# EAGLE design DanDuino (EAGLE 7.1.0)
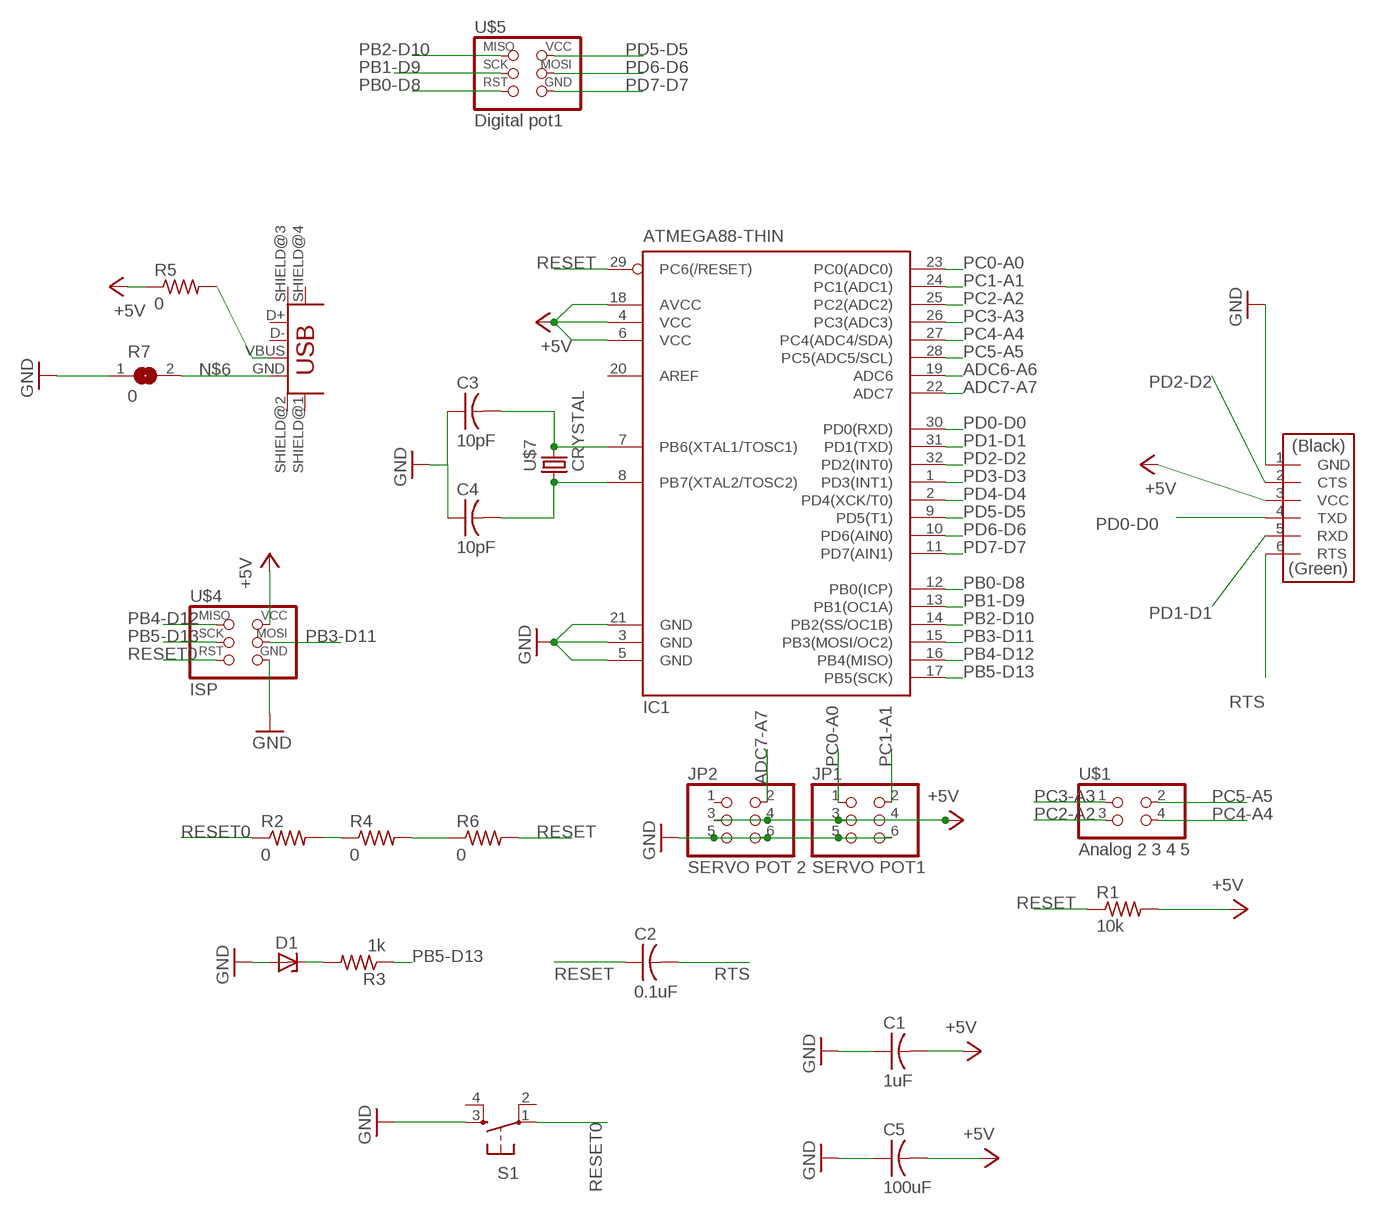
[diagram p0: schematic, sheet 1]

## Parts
C1  1uF  CAP-US1206FAB  [C1206FAB]
C2  0.1uF  CAP-US1206FAB  [C1206FAB]
C3  10pF  CAP-US1206FAB  [C1206FAB]
C4  10pF  CAP-US1206FAB  [C1206FAB]
C5  100uF  CAP-US1206FAB  [C1206FAB]
D1  ZENER_DIODESOD123  [SOD123]
IC1  ATMEGA88-THIN  [TQFP32-08THIN]
JP1  SERVO POT1  PINHD-2X3-SMD  [2X03SMD]
JP2  SERVO POT 2  PINHD-2X3-SMD  [2X03SMD]
R1  10k  RES-US1206FAB  [R1206FAB]
R2  0  RES-US1206FAB  [R1206FAB]
R3  1k  RES-US1206FAB  [R1206FAB]
R4  0  RES-US1206FAB  [R1206FAB]
R5  0  RES-US1206FAB  [R1206FAB]
R6  0  RES-US1206FAB  [R1206FAB]
R7  0  SOLDER_JUMPER  [SJFAB]
S1  6MM_SWITCH6MM_SWITCH  [6MM_SWITCH]
U$1  Analog 2 3 4 5  PINHD-2X2-SMD  [2X02SMD]
U$2  USB_MINIB  [USB_MINIB]
U$3  FTDI-SMD-HEADER  [1X06SMD]
U$4  ISP  AVRISPSMD  [2X03SMD]
U$5  Digital pot1  AVRISPSMD  [2X03SMD]
U$7  CRYSTAL  [2-SMD-5X3MM]

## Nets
+5V: C1.2 C5.2 IC1.4(VCC) IC1.6(VCC) IC1.18(AVCC) JP1.3 JP1.4 JP2.3 JP2.4 R1.2 R5.1 U$3.3(VCC) U$4.2(VCC)
ADC6-A6: IC1.19(ADC6)
ADC7-A7: IC1.22(ADC7) JP2.2
GND: C1.1 C3.1 C4.1 C5.1 D1.ANODE IC1.3(GND) IC1.5(GND) IC1.21(GND) JP1.5 JP1.6 JP2.5 JP2.6 R7.1 S1.3(S) U$3.1(GND) U$4.6(GND)
N$1: C3.2 IC1.7(PB6(XTAL1/TOSC1)) U$7.P$2
N$2: C4.2 IC1.8(PB7(XTAL2/TOSC2)) U$7.P$1
N$3: R4.2 R6.1
N$4: R5.2 U$2.VBUS
N$5: R2.2 R4.1
N$6: R7.2 U$2.GND
N$7: D1.CATHODE R3.2
PB0-D8: IC1.12(PB0(ICP)) U$5.5(RST)
PB1-D9: IC1.13(PB1(OC1A)) U$5.3(SCK)
PB2-D10: IC1.14(PB2(SS/OC1B)) U$5.1(MISO)
PB3-D11: IC1.15(PB3(MOSI/OC2)) U$4.4(MOSI)
PB4-D12: IC1.16(PB4(MISO)) U$4.1(MISO)
PB5-D13: IC1.17(PB5(SCK)) R3.1 U$4.3(SCK)
PC0-A0: IC1.23(PC0(ADC0)) JP1.1
PC1-A1: IC1.24(PC1(ADC1)) JP1.2
PC2-A2: IC1.25(PC2(ADC2)) U$1.3
PC3-A3: IC1.26(PC3(ADC3)) U$1.1
PC4-A4: IC1.27(PC4(ADC4/SDA)) U$1.4
PC5-A5: IC1.28(PC5(ADC5/SCL)) U$1.2
PD0-D0: IC1.30(PD0(RXD)) U$3.4(TXD)
PD1-D1: IC1.31(PD1(TXD)) U$3.5(RXD)
PD2-D2: IC1.32(PD2(INT0)) U$3.2(CTS)
PD3-D3: IC1.1(PD3(INT1))
PD4-D4: IC1.2(PD4(XCK/T0))
PD5-D5: IC1.9(PD5(T1)) U$5.2(VCC)
PD6-D6: IC1.10(PD6(AIN0)) U$5.4(MOSI)
PD7-D7: IC1.11(PD7(AIN1)) U$5.6(GND)
RESET: C2.1 IC1.29(PC6(/RESET)) R1.1 R6.2
RESET0: R2.1 S1.1(P) U$4.5(RST)
RTS: C2.2 U$3.6(RTS)
Unconnected: IC1.20(AREF) JP2.1 S1.2(P1) S1.4(S1) U$2.D+ U$2.D- U$2.SHIELD@1(SHIELD) U$2.SHIELD@2(SHIELD1) U$2.SHIELD@3(SHIELD2) U$2.SHIELD@4(SHIELD3)

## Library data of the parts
C1-C5 = fab:CAP-US
D1 = fab:ZENER_DIODE: zener diode
IC1 = fab:ATMEGA88-THIN
JP1 JP2 = fab:PINHD-2X3-SMD: PIN HEADER
R1-R6 = fab:RES-US: Resistor (US Symbol)
R7 = fab:SOLDER_JUMPER
S1 = fab:6MM_SWITCH: OMRON SWITCH
U$1 = fab:PINHD-2X2-SMD
U$2 = fab:USB_MINIB
U$3 = fab:FTDI-SMD-HEADER
U$4 U$5 = fab:AVRISP
U$7 = fab:CRYSTAL

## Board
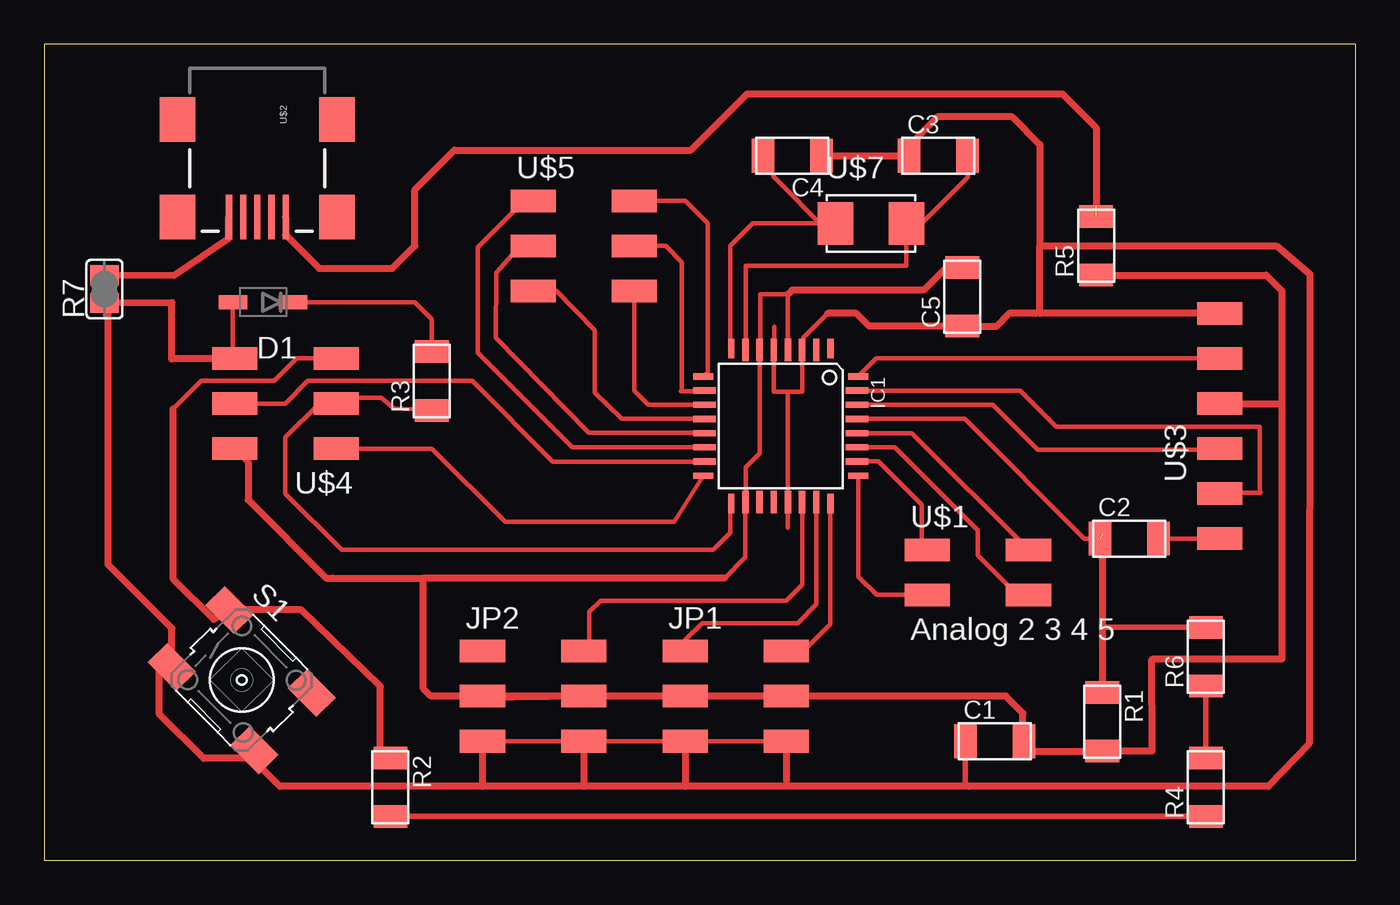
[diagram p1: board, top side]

Size 73.97 x 46.03 mm. Coordinates in mm from the lower left corner, seen from the top.
Outline: 0,0 73.97,0 73.97,46.03 0,46.03 0,0
Copper layers (1*16): Top 0.035mm / dielectric 1.5mm / Bottom 0.035mm
Design rules "default": minimum track width 10mil, minimum drill 24mil, track to track 8mil, track to pad 8mil, pad to pad 8mil, via to via 8mil, smd to smd 8mil, copper to edge 40mil, drill to drill 8mil, minimum pad ring 10mil, minimum via ring 8mil, stop-mask expansion 4mil, vias tented up to drill 0mil, thermal gap 10mil

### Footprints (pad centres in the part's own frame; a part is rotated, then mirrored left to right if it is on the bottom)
C1206FAB = smd 1.27 x 1.905: 1 -1.651,0; 2 1.651,0
SOD123 = smd 1.6 x 0.8: ANODE 1.7,0; CATHODE -1.7,0
TQFP32-08THIN = smd 1.118 x 0.356: 1 -4.369,2.8; 8 -4.369,-2.8; 17 4.369,-2.8; 24 4.369,2.8 | smd 1.27 x 0.356: 2 -4.293,2; 3 -4.293,1.2; 4 -4.293,0.4; 5 -4.293,-0.4; 6 -4.293,-1.2; 7 -4.293,-2; 18 4.293,-2; 19 4.293,-1.2; 20 4.293,-0.4; 21 4.293,0.4; 22 4.293,1.2; 23 4.293,2 | smd 0.356 x 1.118: 9 -2.8,-4.369; 16 2.8,-4.369; 25 2.8,4.369; 32 -2.8,4.369 | smd 0.356 x 1.27: 10 -2,-4.293; 14 1.2,-4.293; 15 2,-4.293; 26 2,4.293; 27 1.2,4.293; 31 -2,4.293 | smd 0.35 x 1.27: 11 -1.2,-4.293; 12 -0.4,-4.293; 13 0.4,-4.293; 28 0.4,4.293; 29 -0.4,4.293; 30 -1.2,4.293
2X03SMD = smd 2.54 x 1.27: 1 -2.857,2.54; 2 2.857,2.54; 3 -2.857,0; 4 2.857,0; 5 -2.857,-2.54; 6 2.857,-2.54
R1206FAB = smd 1.27 x 1.905: 1 -1.651,0; 2 1.651,0
SJFAB = smd 1.118 x 1.6: 1 -0.787,0; 2 0.787,0
6MM_SWITCH = smd 2.286 x 1.524: 1 -3.302,2.286; 2 3.302,2.286; 3 -3.302,-2.286; 4 3.302,-2.286
2X02SMD = smd 2.54 x 1.27: 1 -2.857,1.27; 2 2.857,1.27; 3 -2.857,-1.27; 4 2.857,-1.27
USB_MINIB = smd 2.5 x 0.35: D+ 3.77,0; D- 3.77,0.8; GND 3.77,-1.6; ID 3.77,-0.8; VBUS 3.77,1.6 | smd 2.5 x 2: SHIELD@1 -1.73,-4.5; SHIELD@2 -1.73,4.5; SHIELD@3 3.77,4.5; SHIELD@4 3.77,-4.5
1X06SMD = smd 2.54 x 1.27: 1 0,6.35; 2 0,3.81; 3 0,1.27; 4 0,-1.27; 5 0,-3.81; 6 0,-6.35
2-SMD-5X3MM = smd 2 x 2.4: P$1 -2,0; P$2 2,0

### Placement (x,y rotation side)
C1  53.61,6.72 0 top
C2  61.2,18.15 0 top
C3  50.43,39.74 0 top
C4  42.18,39.74 180 top
C5  51.78,31.79 90 top
D1  12.33,31.48 180 top
IC1  41.54,24.5 270 top
JP1  39,9.26 0 top
JP2  27.57,9.26 0 top
R1  59.68,7.82 270 top
R2  19.52,4.13 270 top
R3  21.86,27.04 90 top
R4  65.52,4.13 90 top
R5  59.32,34.66 90 top
R6  65.52,11.49 90 top
R7  3.39,32.22 90 top
S1  11.14,10.17 314.8 top
U$1  52.65,16.24 0 top
U$2  12.01,40.06 270 top
U$3  66.31,24.5 0 top
U$4  13.6,25.77 180 top
U$5  30.43,34.66 0 top
U$7  46.62,35.93 0 top

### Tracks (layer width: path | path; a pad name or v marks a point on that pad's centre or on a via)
+5V
  Top 0.254: 55.19,6.15 C1.2 | 41.94,31.94 40.37,31.94 40.37,28.79 IC1.6 40.34,22.97 39.56,22.19 39.56,20.22 IC1.18 39.54,17.09 39.46,17.01 39.45,17.01 38.37,15.93 | 41.95,31.94 41.94,31.94 | 41.94,31.94 IC1.4
  Top 0.406: R5.1 68.91,33.01 69.8,32.12 69.8,25.77 | 69.8,25.77 69.8,11.35 62.47,11.34 62.48,6.17 R1.2 59.68,6.15 55.19,6.15 55.19,8.31 54.24,9.26 JP1.4 JP1.3 JP2.4 | U$3.3 69.8,25.77 | JP2.4 JP2.3 | C5.2 50.86,33.44 49.59,32.17 42.18,32.17 41.95,31.94 | 38.37,15.93 21.37,15.93 | JP2.4 24.57,9.18 23.76,9.11 23.61,9.26 21.81,9.26 21.37,9.69 21.37,15.93 | U$4.2 11.49,22.48 11.49,20.33 15.91,15.91 16.24,15.91 16.26,15.93 21.37,15.93
ADC7-A7
  Top 0.254: IC1.22 42.74,15.54 41.86,14.66 31.38,14.66 30.75,14.02 30.75,12.12 JP2.2
GND
  Top 0.254: 63.13,30.85 56.15,30.85 | C3.1 C4.1 | D1.ANODE 10.63,28.42 U$4.6 | JP2.5 JP2.6 JP1.5 JP1.6 | IC1.5 41.14,26.43 41.94,26.43 | 41.94,26.43 42.74,26.43 IC1.3 42.81,28.86 42.81,29.48 44.18,30.85 | 41.94,26.43 IC1.21 41.92,20.21 41.92,18.76 | 55.92,30.85 56.15,31.08 | IC1.5 | IC1.5 41.16,30.09
  Top 0.305: C1.1 51.96,4.38 52.16,4.18
  Top 0.406: 56.15,34.66 56.15,40.37 54.56,41.96 50.43,41.96 48.21,39.74 C4.1 | U$3.1 56.15,30.85 56.15,31.08 56.15,34.66 | 56.15,34.66 69.48,34.66 71.39,33.07 71.34,6.58 69.04,4.18 52.16,4.18 36.14,4.18 | 36.14,4.18 30.43,4.18 | 30.43,4.18 24.71,4.18 | 24.71,4.18 13.28,4.18 11.67,5.79 11.67,5.88 11.54,5.75 8.98,5.75 6.49,8.24 6.49,10.78 6.61,10.9 S1.3 7.19,13.08 3.59,16.68 3.59,31.23 R7.1 7.2,31.46 7.18,28.28 10.49,28.28 10.63,28.42 | JP2.5 24.71,4.18 | JP1.6 41.86,4.5 | JP1.5 36.14,4.18 | JP2.6 30.43,4.18 | 55.92,30.85 54.42,30.85 53.68,30.11 51.8,30.11 C5.1 46.52,30.14 45.81,30.85 44.18,30.85
N$1
  Top 0.254: C3.2 52.08,38.53 49.16,35.61 48.94,35.61 U$7.P$2 48.62,33.54 39.56,33.54 39.56,28.94 IC1.7
N$2
  Top 0.254: C4.2 41.16,38.53 44.08,35.61 44.3,35.61 U$7.P$1 39.95,35.93 38.68,34.66 38.68,28.92 IC1.8
N$3
  Top 0.305: R6.1 R4.2
N$4  (1 unrouted)
  Top 0.406: U$2.VBUS 13.61,35.28 15.51,33.39 19.63,33.39 20.9,34.66 20.9,37.83 23.13,40.06 36.46,40.06 39.64,43.23 57.42,43.23 59.32,41.33 R5.2 | 59.32,36.88 59.96,36.25
N$5
  Top 0.305: R2.2 R4.1
N$6
  Top 0.406: U$2.GND 10.38,36.25 10.38,35.06 7.3,32.98 R7.2
N$7
  Top 0.254: D1.CATHODE 20.9,31.48 21.86,30.53 R3.2
PB0-D8
  Top 0.254: U$5.5 28.87,32.12 31.05,29.91 31.05,26.38 32.58,24.9 IC1.12
PB1-D9
  Top 0.254: U$5.3 26.84,34.66 25.49,33.13 25.46,29.48 30.72,24.12 37.23,24.12 IC1.13
PB2-D10
  Top 0.254: U$5.1 27.06,37.2 24.45,34.58 24.45,28.64 29.78,23.3 IC1.14
PB3-D11
  Top 0.254: U$4.4 13.6,25.77 14.87,27.04 24.14,27.04 28.69,22.49 IC1.15
PB4-D12
  Top 0.254: U$4.1 21.86,23.23 25.98,19.1 35.53,19.1 IC1.16
PB5-D13
  Top 0.254: IC1.17 38.68,20.07 38.68,18.47 37.73,17.51 16.78,17.51 13.6,20.69 13.6,23.86 15.51,25.77 U$4.3 16.78,26.09 19,26.09 19.7,25.51 R3.1
PC0-A0
  Top 0.254: IC1.23 43.54,14.43 42.49,13.39 37.1,13.39 36.14,12.43 JP1.1
PC1-A1
  Top 0.254: IC1.24 44.34,13.33 42.81,11.8 JP1.2
PC2-A2
  Top 0.254: IC1.25 45.91,16 46.94,14.97 U$1.3
PC3-A3
  Top 0.254: IC1.26 47.03,22.5 49.48,20.05 49.48,17.83 U$1.1
PC4-A4
  Top 0.254: IC1.27 47.97,23.3 52.64,18.63 52.64,17.21 55,14.85 55.38,14.85 U$1.4
PC5-A5
  Top 0.254: IC1.28 48.93,24.1 U$1.2
PD0-D0
  Top 0.254: IC1.30 53.5,25.7 56.05,23.15 66.23,23.15 U$3.4
PD1-D1
  Top 0.254: IC1.31 55.04,26.5 57.09,24.45 68.57,24.45 68.57,20.74 | 68.57,20.74 68.62,20.74 | 68.57,20.74 66.31,20.74 U$3.5
PD2-D2
  Top 0.254: U$3.2 46.92,28.31 IC1.32
PD5-D5
  Top 0.254: U$5.2 36.14,37.2 37.41,35.93 37.41,27.54 IC1.9
PD6-D6
  Top 0.254: U$5.4 35.04,34.66 35.95,33.74 35.95,26.5 35.9,26.45 37.2,26.45 IC1.10 37.18,26.43
PD7-D7
  Top 0.254: U$5.6 33.29,26.48 34.07,25.69 IC1.11
RESET  (1 unrouted)
  Top 0.254: 45.92,24.82 IC1.29 51.9,24.9 58.66,18.15 C2.1
  Top 0.305: R6.2 59.86,13.14 59.68,13.32
  Top 0.406: 59.75,18.4 59.68,18.4 59.68,13.32 R1.1
RESET0
  Top 0.254: U$4.5 14.24,28.31 12.97,27.04 8.84,27.04 7.25,25.45
  Top 0.305: 19.49,5.8 R2.1
  Top 0.406: 19.49,5.8 18.96,6.34 18.96,9.82 14.5,14.13 S1.1 9.54,13.6 7.25,15.89 7.25,25.45
RTS
  Top 0.254: C2.2 U$3.6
